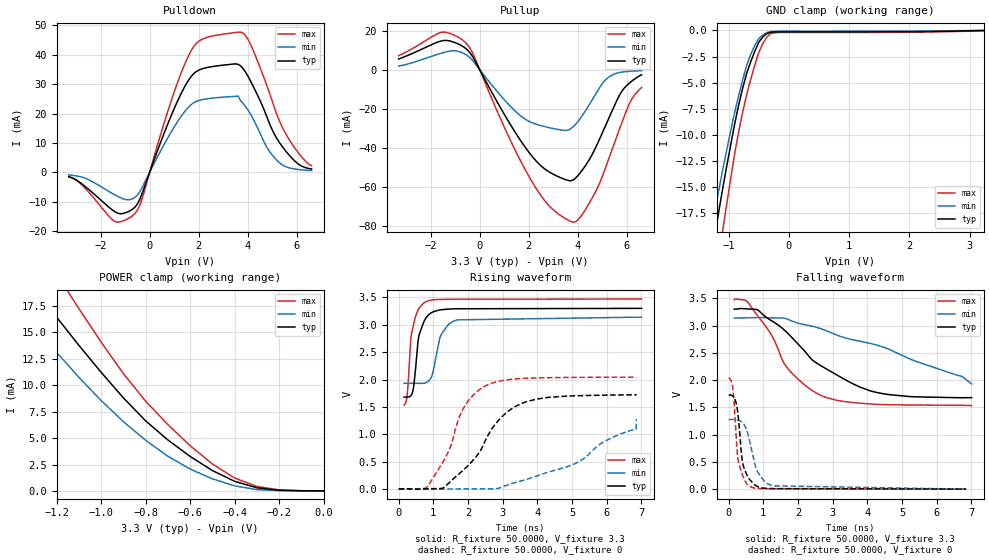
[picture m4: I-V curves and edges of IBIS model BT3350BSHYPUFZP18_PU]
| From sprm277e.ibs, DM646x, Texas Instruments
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| Pin_model   BT3350BSHYPUFZP18_PUon_V33
[Model]   BT3350BSHYPUFZP18_PU
Model_type   I/O
Polarity   Non-Inverting
Enable   Active-Low
Vinl =  0.8V
Vinh =  2V
Cref =  10.0000pF
Rref =  50.0000
Vref =  1.5V
Vmeas =  1.65
C_comp   1.736544p   1.681325p   1.789752p
[Model Spec]
Vinl   0.8V   0.8V   0.8V
Vinh   2V   2V   2V
[Temperature Range]   25   105   0
[Voltage Range]   3.3   3.14   3.47
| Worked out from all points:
|   slope of the pulldown table from 0 to 0.495 V, typ, clamps not added: 44 ohm
|   slope of the pullup table from 0 to 0.495 V, typ, clamps not added: 42.8 ohm
|   GND clamp passes 1 mA (typ) near -0.48 V on its own axis
|   POWER clamp passes 1 mA (typ) near -0.41 V on its own axis
|   rising waveform, R_fixture 50.0000, V_fixture 3.3: 20-80 % time 223ps typ, 309ps min, 188ps max; typ from 1.68 V to 3.3 V
|   rising waveform, R_fixture 50.0000, V_fixture 0: 20-80 % time 1.22ns typ, 2.4ns min, 842ps max; typ from 0.003 V to 1.73 V
|   falling waveform, R_fixture 50.0000, V_fixture 3.3: 20-80 % time 1.88ns typ, 3.36ns min, 1.22ns max; typ from 3.3 V to 1.68 V
|   falling waveform, R_fixture 50.0000, V_fixture 0: 20-80 % time 204ps typ, 351ps min, 171ps max; typ from 1.73 V to 0.003 V
[POWER_clamp]
|   voltage   I(typ)   I(min)   I(max)
-3.3V     86.16mA    67.13mA    105mA
-1.433V   23.25mA    19mA       28.67mA
-1.4V     22.2mA     18.14mA    27.44mA
-1.267V   18.31mA    14.78mA    22.82mA
-1.133V   14.68mA    11.55mA    18.37mA
-900mV    8.817mA    6.569mA    11.11mA
-800mV    6.639mA    4.799mA    8.503mA
-700mV    4.827mA    3.28mA     6.281mA
-500mV    1.929mA    1.146mA    2.549mA
-400mV    907.2uA    478uA      1.218mA
-300mV    294.5uA    124.1uA    421.8uA
0V        111.6nA    122.2nA    531.1nA
[Pulldown]
|   voltage   I(typ)   I(min)   I(max)
-3.3V     -1.512mA   -878.6uA   -1.478mA
-1.4V     -13.5mA    -7.754mA   -16.8mA
-700mV    -12.58mA   -9.011mA   -14.79mA
-400mV    -9.19mA    -6.568mA   -11.22mA
900mV     19.74mA    14.05mA    24.87mA
1.7V      32.7mA     23.1mA     41.52mA
2.2V      35.39mA    24.85mA    45.53mA
3.6V      36.79mA    25.98mA    47.71mA
4.1V      31.25mA    19.99mA    43.72mA
5.2V      11.29mA    3.971mA    19.31mA
5.8V      4.817mA    1.297mA    9.688mA
6.6V      1.129mA    610.1uA    2.216mA
[Pullup]
|   voltage   I(typ)   I(min)   I(max)
-3.3V     5.397mA    1.812mA    7.127mA
-1.6V     14.52mA    8.233mA    18.96mA
-600mV    11.14mA    7.955mA    14.14mA
-300mV    6.902mA    4.842mA    8.811mA
1.3V      -29.12mA   -19.41mA   -37.45mA
2.2V      -45.34mA   -27.5mA    -58.77mA
2.9V      -52.91mA   -29.94mA   -70.62mA
3.8V      -56.6mA    -29.4mA    -78.14mA
4.5V      -45.44mA   -17.28mA   -67.66mA
5.2V      -26.74mA   -4.474mA   -47.85mA
6.1V      -6.94mA    -895.2uA   -17.5mA
6.6V      -2.652mA   -585.1uA   -9.182mA
[GND_clamp]
|   voltage   I(typ)   I(min)   I(max)
-3.3V     -101.9mA   -80.83mA   -121.5mA
-1.3V     -22.23mA   -19.42mA   -27.13mA
-1.233V   -19.8mA    -17.39mA   -24.45mA
-1.167V   -17.45mA   -15.39mA   -21.82mA
-1.1V     -15.2mA    -13.41mA   -19.23mA
-1.033V   -13.07mA   -11.5mA    -16.71mA
-900mV    -8.978mA   -7.863mA   -11.83mA
-700mV    -4.111mA   -3.334mA   -6.141mA
-500mV    -1.141mA   -794.5uA   -2.129mA
-366.7mV  -309.2uA   -210.5uA   -650.5uA
-166.7mV  -140.6uA   -75.05uA   -198.7uA
3.233V    -8.733uA   9.396uA    -38.37uA
[Ramp]
| variable   typ   min   max
dV/dt_f   0.984392/1.9018313n 0.76805453/3.5496673n  1.1728981/1.2350833n
dV/dt_r  1.0409375/1.2292146n 0.77628069/2.4455528n  1.2301703/0.84780407n
R_load = 50
[Rising Waveform]
R_fixture = 50.0000
V_fixture = 3.3
V_fixture_min = 3.14
V_fixture_max = 3.47
|   time   V(typ)   V(min)   V(max)
158.4ps   1.68V      1.93V      1.535V
247.4ps   1.681V     1.931V     1.73V
379.4ps   1.731V     1.931V     2.865V
438.3ps   1.895V     1.931V     3.021V
580ps     2.779V     1.931V     3.29V
801.3ps   3.136V     1.945V     3.426V
976.5ps   3.23V      2.102V     3.455V
1.226ns   3.274V     2.818V     3.464V
1.69ns    3.293V     3.09V      3.467V
7.008ns   3.3V       3.14V      3.47V
[Rising Waveform]
R_fixture = 50.0000
V_fixture = 0
V_fixture_min = 0
V_fixture_max = 0
|   time   V(typ)   V(min)   V(max)
2.236ps   3.146mV    1.93mV     3.847mV
826.7ps   4.911mV    1.344mV    41.58mV
1.411ns   85.98mV    353.6uV    650.1mV
1.915ns   375.2mV    3.413mV    1.525V
2.548ns   944.8mV    3.815mV    1.899V
3.096ns   1.388V     64.44mV    1.991V
3.763ns   1.61V      191.1mV    2.025V
5.214ns   1.706V     506.2mV    2.04V
6.85ns    1.721V     1.099V     2.044V
6.852ns   1.732V     1.277V     2.046V
[Falling Waveform]
R_fixture = 50.0000
V_fixture = 3.3
V_fixture_min = 3.14
V_fixture_max = 3.47
|   time   V(typ)   V(min)   V(max)
158.4ps   3.3V       3.14V      3.47V
506.2ps   3.307V     3.142V     3.457V
857.7ps   3.279V     3.148V     3.162V
1.244ns   3.087V     3.142V     2.819V
1.692ns   2.868V     3.12V      2.226V
2.191ns   2.534V     3.018V     1.914V
2.651ns   2.268V     2.946V     1.724V
4.277ns   1.774V     2.643V     1.557V
6.749ns   1.678V     2.063V     1.539V
7.008ns   1.68V      1.93V      1.535V
[Falling Waveform]
R_fixture = 50.0000
V_fixture = 0
V_fixture_min = 0
V_fixture_max = 0
|   time   V(typ)   V(min)   V(max)
2.236ps   1.732V     1.277V     2.046V
84.64ps   1.722V     1.279V     1.971V
129.1ps   1.703V     1.278V     1.813V
241.5ps   1.5V       1.271V     737mV
276.7ps   1.338V     1.265V     532.2mV
403.4ps   493.2mV    1.219V     256.1mV
594.2ps   186.6mV    921.7mV    54.7mV
829.9ps   52.15mV    329.2mV    15.68mV
1.274ns   12.09mV    63.13mV    8.24mV
6.852ns   3.146mV    1.93mV     3.847mV
